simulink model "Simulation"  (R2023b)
settings: Solver=ode23t  StartTime=0.0  StopTime=10  RelTol=1e-3  EnableMultiTasking=on
libraries: fl_lib x7, nesl_utility x3, batteryecm_lib x1, ee_lib x1, sdl_lib x1

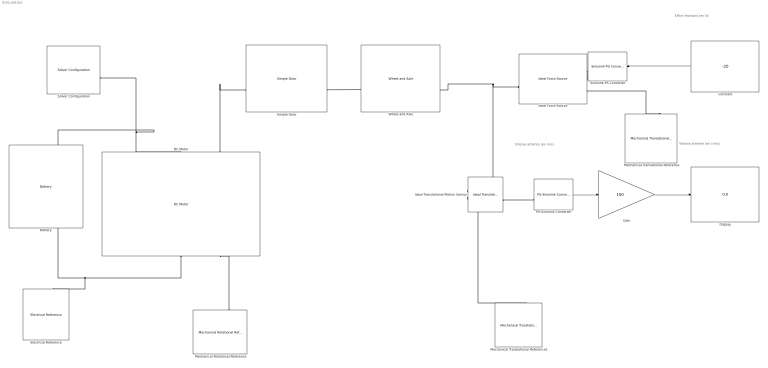
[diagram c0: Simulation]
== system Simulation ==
  note: Effort résistant (en N)
  note: Vitesse atteinte (en cm/s)
  note: Vitesse atteinte (en m/s)
  Battery : batteryecm_lib/Battery  Vnom=3.7 V  prm_dir=simscape.enum.battery.prm_dir.disabled  R1_dis=2 Ohm  R1_ch=2 Ohm  R1=0.1 Ohm  prm_AH=1  AH=50 hr*A  V1=11.5 V  AH1=25 hr*A  prm_R2=1  R2=2e+3 Ohm  Tmeas=298.15 K  charge_measurement_port=simscape.enum.battery.enable.no  prm_dyn=simscape.enum.battery.prm_dyn.off  Rp1=0.005 Ohm  tau1=30 s  Rp2=0.005 Ohm  tau2=30 s  Rp3=0.005 Ohm  tau3=30 s  Rp4=0.005 Ohm  tau4=30 s  Rp5=0.005 Ohm  tau5=30 s  prm_fade=1  N_fade=100  AH_fade=45 hr*A  R1_fade=2.02 Ohm  R1_ch_fade=2.02 Ohm  V1_fade=10.35 V  prm_age=simscape.enum.battery.prm_age.disabled  prm_age_OCV=simscape.enum.battery.prm_age_OCV.OCV  OCV_age=0.9  SOC_age=60  Tmeas_age=298.15 K  delta_time_age_vec=[0] d  temperature_age_vec=[273] K  OCV_scaling_age=2.2134e6  OCV_offset_age=1.632e6  temp_exp_age=0.515833569 V  t_exp_age=0.75  Vnom_T2=12 V  R1_T2=2.2 Ohm  R1_T2_dis=2.2 Ohm  R1_T2_ch=2.2 Ohm  V1_T2=11.4 V  R2_T2=2200 Ohm  Rp1_T2=0.005 Ohm  tau1_T2=30 s  Rp2_T2=0.005 Ohm  tau2_T2=30 s  Rp3_T2=0.005 Ohm  tau3_T2=30 s  Rp4_T2=0.005 Ohm  tau4_T2=30 s  Rp5_T2=0.005 Ohm  tau5_T2=30 s  Tmeas2=273.15 K  thermal_port=simscape.enum.thermaleffects.omit  thermal_mass=30000 J/K  i_specify=off  i_priority=None  i=0 A  i_nominal_specify=off  i_nominal_unit=A  i_nominal_value=1  v_specify=off  v_priority=None  v=0 V  v_nominal_specify=off  v_nominal_unit=V  v_nominal_value=1  charge_specify=on  charge_priority=High  charge=50 hr*A  charge_nominal_specify=off  charge_nominal_unit=A*hr  charge_nominal_value=1  num_cycles_specify=off  num_cycles_priority=High  num_cycles=0  num_cycles_nominal_specify=off  num_cycles_nominal_unit=1  num_cycles_nominal_value=1  temperature_specify=off  temperature_priority=High  temperature=298.15 K  temperature_nominal_specify=off  temperature_nominal_unit=K  temperature_nominal_value=1
  Constant : Constant  Value=-20
  DC Motor : ee_lib/Electromechanical/Brushed Motors/DC Motor  field_option=ee.enum.field_option.pm  Rf=100 Ohm  Lf=1 H  Laf=0.15 H  If0=0 A  parameterization=2  Ra=3.9 Ohm  La=1.2e-5 H  emf_or_torque=1  Kv=7.2e-5 V/rpm  Ki=6.876e-4 N*m/A  T_stall=0.777 N*m  w_max=9000 rpm  w_rated=5950 rpm  P_rated=7 W  V_rated=5 V  lam_param=2  i_noload=0.035 A  V_i_noload=3.9 V  J=0.01 g*cm^2  lam=0 N*m/(rad/s)  speed0=0 rpm  enable_fault_armature=simscape.enum.onoff.off  rev_faulted=1 / 3  G_faulted_armature=1e-5 S  fault_trigger_armature=ee.enum.faults.faultTrigger.temporal  t_fault_armature=1 s  max_permissible_current_armature=inf A  t_fail_on_current_armature=1 s  enable_fault_field=simscape.enum.onoff.off  G_faulted_field=1e-5 S  fault_trigger_field=ee.enum.faults.faultTrigger.temporal  t_fault_field=1 s  max_permissible_current_field=inf A  t_fail_on_current_field=1 s  fault_action=simscape.enum.assert.action.none  alpha=3.93e-3 1/K  Tmeas=25 degC  thermal_mass=100 J/K  initial_temperature=25 degC
  Display : Display
  Electrical Reference : fl_lib/Electrical/Electrical Elements/Electrical Reference
  Gain : Gain  Gain=100
  Ideal Force Source : fl_lib/Mechanical/Mechanical Sources/Ideal Force Source
  Ideal Translational Motion Sensor : fl_lib/Mechanical/Mechanical Sensors/Ideal Translational Motion Sensor  reference=foundation.enum.MeasurementReference.difference  acceleration_port=false  velocity_port=true  position_port=true  offset=0 m
  Mechanical Rotational Reference : fl_lib/Mechanical/Rotational Elements/Mechanical Rotational Reference
  Mechanical Translational Reference : fl_lib/Mechanical/Translational Elements/Mechanical Translational Reference
  Mechanical Translational Reference1 : fl_lib/Mechanical/Translational Elements/Mechanical Translational Reference
  PS-Simulink Converter : nesl_utility/PS-Simulink Converter  PhysicalDomain=network_engine_domain  SubClassName=ps_output  LeftPortType=input  RightPortType=output  PseudoPeriodic=off  Frequencies=[]  VectorFormat=1-D array  Unit=1  AffineConversion=off
  Simple Gear : sdl_lib/Gears/Simple Gear  ratio=0  rotation_direction=3-2*(1)  friction_model=2  T_noload=0.1 N*m  T_nom=5 N*m  efficiency_nom=0.8  efficiency=0.81  temperature_TLU=[280.0, 300.0, 320.0] K  load_TLU=[1.0, 5.0, 10.0] N*m  efficiency_TLU=[0.95, 0.9, 0.85]  efficiency_TLU2=[0.85, 0.8, 0.75; 0.95, 0.9, 0.85; 0.85, 0.8, 0.7]  w_thr=0.01 rad/s  pwr_thr=0.001 W  enable_backlash=false  hardstop_model=simscape.enum.hardstop.smooth  backlash_distance=1e-3 mm  r_base=0.1 m  transition=1e-4 mm  backlash_stiffness=1e6 N/m  backlash_damping=1e3 N*s/m  coeff_rest=0.7  v_tol=0.001 m/s  f_tol=0 N  mu_visc=[0.0, 0.0] N*m/(rad/s)  enable_faults=simscape.enum.onoff.off  efficiency_fault=0.05  external_fault=simscape.enum.onoff.off  temporal_fault=simscape.enum.onoff.off  fault_time=5 s  fault_angles=pi / 12 rad  report_fault=simscape.enum.assert.action.none  thermal_mass=50 J/K  temperature_specify=off  temperature_priority=High  temperature=300 K  temperature_nominal_specify=off  temperature_nominal_unit=K  temperature_nominal_value=1  x_backlash_specify=off  x_backlash_priority=None  x_backlash=0 mm  x_backlash_nominal_specify=off  x_backlash_nominal_unit=mm  x_backlash_nominal_value=1  f_hardstop_specify=off  f_hardstop_priority=None  f_hardstop=0 N  f_hardstop_nominal_specify=off  f_hardstop_nominal_unit=N  f_hardstop_nominal_value=1  v_backlash_specify=off  v_backlash_priority=None  v_backlash=0 m/s  v_backlash_nominal_specify=off  v_backlash_nominal_unit=m/s  v_backlash_nominal_value=1
  Simulink-PS Converter : nesl_utility/Simulink-PS Converter  PhysicalDomain=network_engine_domain  SubClassName=ps_input  LeftPortType=input  RightPortType=output  PseudoPeriodic=off  Frequencies=[]  NoiseDistribution=none  NoiseParameters=[]  Unit=1  AffineConversion=off  FilteringAndDerivatives=zero  SimscapeFilterOrder=1  InputFilterTimeConstant=0.001  UdotUserProvided=1
  Solver Configuration : nesl_utility/Solver Configuration  PhysicalDomain=network_engine_domain  SubClassName=solver  LeftPortType=input  RightPortType=generic  Tones=[]  Harmonics=[]  SimulateNoise=off  Profile=off  UseLocalSampling=off  EnableSwitchedLinearOptims=on  FrequencyDomain=off  UseCCode=off  RelTol=0.001  AbsTol=1e-06  MinStep=1e-09  ToWorkspace=off  RevertToSquareIcSolve=off  NumHomotopyIterations=100  PhasorMode=off  PhasorModeNumHarmonics=1  ConsistencySolver=NEWTON_FTOL  IndexReductionMethod=DerivativeReplacement  DoDC=off  ResidualTolerance=1e-09  ConsistencyTolSource=GLOBAL  ConsistencyAbsTol=0.001  ConsistencyRelTol=0.001  ConsistencyTolFactor=0.001  UseLocalSolver=off  LocalSolverChoice=NE_BACKWARD_EULER_ADVANCER  ResolveIndetEquations=on  FunctionEvalNumThread=1  LocalSolverSampleTime=0.001  DoFixedCost=off  MaxNonlinIter=3  MaxModeIter=2  ComputeImpulses=off  ImpulseIterations=2  LinearAlgebra=Sparse  LinearAlgebraNumThread=0  EquationFormulation=NE_TIME_EF  DelaysMemoryBudget=1024  AutomaticFiltering=on  FilteringTimeConstant=0.001  PartitionStorageMethod=AS_NEEDED  PartitionMemoryBudget=1024  PartitionMethod=FAST  MultibodyUseLocalSolver=off  MultibodyLocalSolverChoice=ODE1  MultibodyLocalSolverSampleTime=0.001
  Wheel and Axle : fl_lib/Mechanical/Mechanisms/Wheel and Axle  R=18.5 mm  or=1  t_specify=off  t_priority=None  t=0 N*m  t_nominal_specify=off  t_nominal_unit=N*m  t_nominal_value=1  f_specify=off  f_priority=None  f=0 N  f_nominal_specify=off  f_nominal_unit=N  f_nominal_value=1
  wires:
  Constant/1 -> Simulink-PS Converter/1
  PS-Simulink Converter/1 -> Gain/1
  Gain/1 -> Display/1
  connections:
  DC Motor/RConn1 -- Battery/RConn1 -- Electrical Reference/LConn1
  Ideal Translational Motion Sensor/RConn1 -- Mechanical Translational Reference1/LConn1
  Solver Configuration/RConn1 -- Battery/LConn1 -- DC Motor/LConn1
  Ideal Force Source/RConn2 -- Mechanical Translational Reference/LConn1
  Ideal Translational Motion Sensor/LConn1 -- Ideal Force Source/LConn1 -- Wheel and Axle/RConn1
  Mechanical Rotational Reference/LConn1 -- DC Motor/RConn2
  DC Motor/LConn2 -- Simple Gear/LConn1
  Simple Gear/RConn1 -- Wheel and Axle/LConn1
  Simulink-PS Converter/RConn1 -- Ideal Force Source/RConn1
  Ideal Translational Motion Sensor/RConn2 -- PS-Simulink Converter/LConn1
